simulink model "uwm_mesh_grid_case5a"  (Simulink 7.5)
settings: Solver=ode45  StartTime=0.0  StopTime=3.0  RelTol=1e-4
undefined symbols (not defined in the file or in its folder): D1, Delta, dfilt, DiscIntNeverNeededParam, Discrete, no, powergui, steady, ZData
libraries: powerlib x259, powerlib_extras x68, dsparch4 x11
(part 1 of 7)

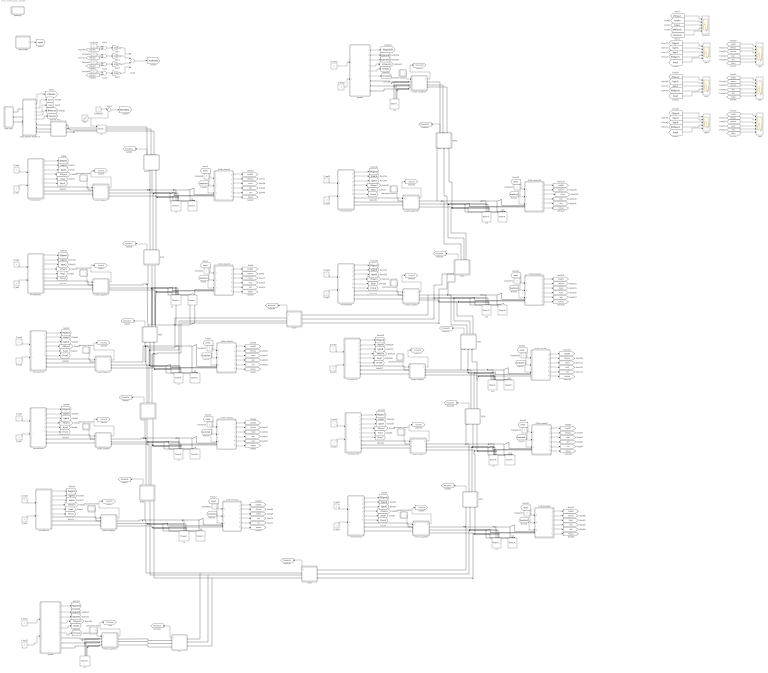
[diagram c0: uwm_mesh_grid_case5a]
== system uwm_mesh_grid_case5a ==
  2 kW e-board5 : Subsystem
  2 kW e-board9 : Subsystem
  4 kW e-board1 : Subsystem
  4 kW e-board10 : Subsystem
  4 kW e-board2 : Subsystem
  4 kW e-board3 : Subsystem
  4 kW e-board4 : Subsystem
  4 kW e-board6 : Subsystem
  4 kW e-board7 : Subsystem
  4 kW e-board8 : Subsystem
  Constant{1..3,9..15} (10 alike) : Constant  Value=2  OutDataType=fixdt(1, 16)  OutScaling=2^0
  Constant{4..8} (5 alike) : Constant  OutDataType=fixdt(1, 16)  OutScaling=2^0
  EB1 : Scope  NumInputPorts=6
  EB5 : Scope  NumInputPorts=6
  EBA : Scope  NumInputPorts=6
  E_req{1,3,5,7,9} (5 alike) : Constant  Value=.3  OutDataType=fixdt(1, 16)  OutScaling=2^0
  E_req{2,4,6,8,10,12,14,16,18,20..22} (12 alike) : Constant  OutDataType=fixdt(1, 16)  OutScaling=2^0
  E_req{11,13,15,17,19} (5 alike) : Constant  Value=.2  OutDataType=fixdt(1, 16)  OutScaling=2^0
  E_req23 : Constant  Value=.8  OutDataType=fixdt(1, 16)  OutScaling=2^0
  E_req24 : Constant  Value=.8  OutDataType=fixdt(1, 16)  OutScaling=2^0
  Gain{,1..3} (4 alike) : Gain  Gain=2/15  ParameterDataType=fixdt(1, 16)  ParameterScaling=2^0  OutDataType=fixdt(1, 16)  OutScaling=2^0
  L{1..20} (20 alike) : powerlib/Elements/Three-Phase Series RLC Load  DialogController=POWERSYS.PowerSysDialog  PhysicalDomain=powersysdomain  SubClassName=unknown  LeftPortType=p1  RightPortType=p1  LConnTagsString=A|B|C  Configuration=Y (grounded)  NominalVoltage=208  NominalFrequency=60  ActivePower=4000  InductivePower=0  CapacitivePower=0  Measurements=None
  L21 : powerlib/Elements/Three-Phase Series RLC Load  DialogController=POWERSYS.PowerSysDialog  PhysicalDomain=powersysdomain  SubClassName=unknown  LeftPortType=p1  RightPortType=p1  LConnTagsString=A|B|C  Configuration=Y (grounded)  NominalVoltage=208  NominalFrequency=60  ActivePower=8000  InductivePower=0  CapacitivePower=0  Measurements=None
  L22 : powerlib/Elements/Three-Phase Series RLC Load  DialogController=POWERSYS.PowerSysDialog  PhysicalDomain=powersysdomain  SubClassName=unknown  LeftPortType=p1  RightPortType=p1  LConnTagsString=A|B|C  Configuration=Y (grounded)  NominalVoltage=208  NominalFrequency=60  ActivePower=8000  InductivePower=0  CapacitivePower=0  Measurements=None
  MainGrid : Scope  NumInputPorts=5
  PC01 : Subsystem  mask{R=0.027352, L=.006600, C=288.6}
  PC1 : Subsystem  mask{R=0.027352, L=.006600, C=288.6}
  PC12 : Subsystem  mask{R=0.027352, L=.006600, C=288.6}
  PC2 : Subsystem  mask{R=.002810, L=.000679, C=2894.3}
  PC23 : Subsystem  mask{R=0.027352, L=.006600, C=288.6}
  PC34 : Subsystem  mask{R=0.027352, L=.006600, C=288.6}
  PC39 : Subsystem  mask{R=0.027352, L=.006600, C=288.6}
  PC45 : Subsystem  mask{R=0.027352, L=.006600, C=288.6}
  PC56 : Subsystem  mask{R=0.027352, L=.006600, C=288.6}
  PC67 : Subsystem  mask{R=0.027352, L=.006600, C=288.6}
  PC78 : Subsystem  mask{R=0.027352, L=.006600, C=288.6}
  PC89 : Subsystem  mask{R=0.027352, L=.006600, C=288.6}
  PC9A : Subsystem  mask{R=0.027352, L=.006600, C=288.6}
  PC9A1 : Subsystem  mask{R=0.027352, L=.006600, C=288.6}
  SS : powerlib/Elements/Three-Phase Breaker  DialogController=POWERSYS.PowerSysDialog  SystemSampleTime=-1  InitialState=closed  SwitchA=on  SwitchB=on  SwitchC=on  SwitchTimes=[1.]  External=on  BreakerResistance=.001  SnubberResistance=1e6  SnubberCapacitance=inf  Measurements=None
  Step : Step  Time=2  Before=1  After=0  SampleTime=0
  Sum{1..3,5} (4 alike) : Sum  Inputs=+-  OutDataType=fixdt(1, 16)  OutScaling=2^0
  Sum4 : Sum  Inputs=|+-  OutDataType=fixdt(1, 16)  OutScaling=2^0
  Sum6 : Sum  Inputs=++++  OutDataType=fixdt(1, 16)  OutScaling=2^0
  disconnect event : Subsystem  mask{tstart=50, tstop=60}
      mask prompts: tstart "disconnect time"; tstop "connect time"
  disconnect event1 : Subsystem  mask{tstart=100, tstop=200}
      mask prompts: tstart "disconnect time"; tstop "connect time"
  disconnect event10 : Subsystem  mask{tstart=100, tstop=200}
      mask prompts: tstart "disconnect time"; tstop "connect time"
  disconnect event11 : Subsystem  mask{tstart=50, tstop=60}
      mask prompts: tstart "disconnect time"; tstop "connect time"
  disconnect event2 : Subsystem  mask{tstart=100, tstop=200}
      mask prompts: tstart "disconnect time"; tstop "connect time"
  disconnect event3 : Subsystem  mask{tstart=100, tstop=200}
      mask prompts: tstart "disconnect time"; tstop "connect time"
  disconnect event4 : Subsystem  mask{tstart=100, tstop=200}
      mask prompts: tstart "disconnect time"; tstop "connect time"
  disconnect event5 : Subsystem  mask{tstart=100, tstop=200}
      mask prompts: tstart "disconnect time"; tstop "connect time"
  disconnect event6 : Subsystem  mask{tstart=100, tstop=200}
      mask prompts: tstart "disconnect time"; tstop "connect time"
  disconnect event7 : Subsystem  mask{tstart=100, tstop=200}
      mask prompts: tstart "disconnect time"; tstop "connect time"
  disconnect event8 : Subsystem  mask{tstart=100, tstop=200}
      mask prompts: tstart "disconnect time"; tstop "connect time"
  disconnect event9 : Subsystem  mask{tstart=100, tstop=200}
      mask prompts: tstart "disconnect time"; tstop "connect time"
  gen1 : Scope  NumInputPorts=5
  gen5 : Scope  NumInputPorts=5
  genA : Scope  NumInputPorts=5
  genset : Subsystem
  genset1 : Subsystem
  main grid : Subsystem
  measurement feeder C3 : Subsystem
  microsource : Subsystem  AncestorBlock=|
      | UWM_blocks/inverter-based
      | DG (simplified)
      | 208V - 15kVA
  microsource1 : Subsystem  AncestorBlock=|
      | UWM_blocks/inverter-based
      | DG (simplified)
      | 208V - 15kVA
  microsource2 : Subsystem  AncestorBlock=|
      | UWM_blocks/inverter-based
      | DG (simplified)
      | 208V - 15kVA
  microsource3 : Subsystem  AncestorBlock=|
      | UWM_blocks/inverter-based
      | DG (simplified)
      | 208V - 15kVA
  microsource4 : Subsystem  AncestorBlock=|
      | UWM_blocks/inverter-based
      | DG (simplified)
      | 208V - 15kVA
  microsource5 : Subsystem  AncestorBlock=|
      | UWM_blocks/inverter-based
      | DG (simplified)
      | 208V - 15kVA
  microsource6 : Subsystem  AncestorBlock=|
      | UWM_blocks/inverter-based
      | DG (simplified)
      | 208V - 15kVA
  microsource7 : Subsystem  AncestorBlock=|
      | UWM_blocks/inverter-based
      | DG (simplified)
      | 208V - 15kVA
  microsource8 : Subsystem  AncestorBlock=|
      | UWM_blocks/inverter-based
      | DG (simplified)
      | 208V - 15kVA
  microsource9 : Subsystem  AncestorBlock=|
      | UWM_blocks/inverter-based
      | DG (simplified)
      | 208V - 15kVA
  powergui : Subsystem  Priority=1  AncestorBlock=powerlib/powergui  InitFcn=powergui( 'InitFcn_Callback' , gcb , 0 , [ ] );  StopFcn=powergui( 'StopFcn_Callback' , gcb , 0 , [ ] );  mask(PSB option menu block){SimulationMode=Discrete, SampleTime=20e-6, frequency=60, SPID=off, DisableSnubberDevices=off, DisableRonSwitches=off, DisableVfSwitches=off, SwTol=0, Interpol=off, frequencyindice=60, echomessages=off, HookPort=off, DisplayEquations=off, FunctionMessages=off, EnableUseOfTLC=off, x0status=steady, RestoreLinks=no, ResistiveCurrentMeasurement=off, Frange=[0:2:500], Ylog=off, Xlog=on, ShowGrid=off, save=off, variable=ZData, structure=, ZoomFFT=on, StartTime=0.0, cycles=1, DisplayStyle=1, fundamental=60, FreqAxis=off, MaxFrequency=1000, frequencyindicesteady=1, RmsSteady=2, display=off, Ts=0, methode=off}
      mask prompts: SimulationMode "Simulation type:"; SampleTime "Sample time (s):"; frequency "Phasor frequency (Hz):"; SPID "Enable use of ideal switching devices"; DisableSnubberDevices "Disable snubbers in switching devices"; DisableRonSwitches "Disable On resistance in switching devices (Ron=0)"; DisableVfSwitches "Disable Forward voltage in switching devices (Vf=0)"; SwTol "Switch tolerance"; Interpol "Interpolate"; frequencyindice "Load flow frequency (Hz):"; echomessages "Display SimPowerSystems warnings and messages"; HookPort "Add a hook port to the powergui block"; DisplayEquations "Display circuit differential equations"; FunctionMessages "Display internal function messages (debug mode feature)"; EnableUseOfTLC "Use TLC file when in Accelerator Simulation Mode and for RTW applications"; x0status "Start simulation with initial electrical states from:"; RestoreLinks "Restore disabled links of SimPowerSystems blocks:"; ResistiveCurrentMeasurement "Use non ideal current measurement blocks (1e-4Ohm internal resistance)"; Frange "Frequency Range"; Ylog "Log impedance"; Xlog "log Frequency"; ShowGrid "grid"; save "Save Data To Workspace"; variable "Variable Name"; structure "Structure Name (PSBFFTSCOPE)"; ZoomFFT "ZoomFFT (PSBFFTSCOPE)"; StartTime "Start Time (PSBFFTSCOPE)"; cycles "Cycles (PSBFFTSCOPE)"; DisplayStyle "Display style (PSBFFTSCOPE)"; fundamental "Fundamental (PSBFFTSCOPE)"; FreqAxis "Frequency Axis (PSBFFTSCOPE)"; MaxFrequency "Max Frequency (PSBFFTSCOPE)"; frequencyindicesteady "Frequency indice (STEADYSTATE)"; RmsSteady "RMS display (STEADYSTATE)"; display "Display Results"; Ts "Old Ts setting (OBSOLETE)"; methode "Phasor simulation (OBSOLETE)"
      mask help: Set simulation type, simulation parameters, and preferences
      mask init:
      | message = powergui('MaskInitialization',gcb,SimulationMode,SampleTime);
  reset pulses : Subsystem  mask{tpulse=[50 100]}
  smart coupler1 : Subsystem
  smart coupler10 : Subsystem
  smart coupler11 : Subsystem
  smart coupler12 : Subsystem
  smart coupler2 : Subsystem
  smart coupler3 : Subsystem
  smart coupler4 : Subsystem
  smart coupler5 : Subsystem
  smart coupler6 : Subsystem
  smart coupler7 : Subsystem
  smart coupler8 : Subsystem
  smart coupler9 : Subsystem
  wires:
  E_req1/1 -> microsource/2(P_req)
  E_req2/1 -> microsource/1(E_req)
  reset pulses/1(Out1) -> [reset]
  4 kW e-board1/1(w) -> [freqEB1]
  4 kW e-board1/2(state) -> [EB1state]
  measurement feeder C3/3(I) -> [Imain]
  measurement feeder C3/1(PQ) -> [PQmain]
  measurement feeder C3/2(V) -> [Vmain]
  [PQmain] -> MainGrid/1
  [Vmain] -> MainGrid/2
  [Imain] -> MainGrid/3
  [RMSmain] -> MainGrid/4
  microsource/1(PQ) -> [PQgen1]
  microsource/2(V) -> [Vgen1]
  microsource/3(I) -> [Igen1]
  microsource/5(freq) -> [freq1]
  measurement feeder C3/4(RMS) -> [RMSmain]
  microsource/4(RMS) -> [RMSgen1]
  measurement feeder C3/5(freq) -> [freqmain]
  [freqmain] -> MainGrid/5
  [freqEB1] -> EB1/1
  [RMSeb1] -> EB1/2
  [EB1state] -> EB1/3
  4 kW e-board1/3(PQ) -> [PQeb1]
  4 kW e-board1/4(V) -> [Veb1]
  4 kW e-board1/5(I) -> [Ieb1]
  4 kW e-board1/6(RMS) -> [RMSeb1]
  [PQeb1] -> EB1/6
  [Ieb1] -> EB1/5
  [Veb1] -> EB1/4
  Step/1 -> SS/1, Sum4/2
  Constant5/1 -> Sum4/1
  Sum4/1 -> [IslandState]
  disconnect event1/1(Out1) -> smart coupler1/1(event)
  smart coupler1/1(connected) -> [connect1]
  Constant4/1 -> Sum1/1
  [EB1state] -> Sum1/2
  Constant6/1 -> Sum2/1
  [EB2state] -> Sum2/2
  Constant7/1 -> Sum3/1
  [EB3state] -> Sum3/2
  Constant8/1 -> Sum5/1
  [EB4state] -> Sum5/2
  Sum1/1 -> Gain/1
  Sum2/1 -> Gain1/1
  Sum3/1 -> Gain3/1
  Sum5/1 -> Gain2/1
  Gain1/1 -> Sum6/2
  Gain3/1 -> Sum6/3
  Gain/1 -> Sum6/1
  Gain2/1 -> Sum6/4
  Sum6/1 -> [loadshed]
  [reset] -> 4 kW e-board1/1(reset)
  Constant9/1 -> 4 kW e-board1/2(priority)
  [loadshed] -> 4 kW e-board1/3(shed_load)
  PC01/1(PQ) -> [PQcable01]
  microsource/6(Pmm) -> [Pmm1]
  [PQgen1] -> gen1/1
  [Vgen1] -> gen1/2
  [Igen1] -> gen1/3
  [RMSgen1] -> gen1/4
  [freq1] -> gen1/5
  E_req3/1 -> microsource1/2(P_req)
  E_req4/1 -> microsource1/1(E_req)
  4 kW e-board2/1(w) -> [freqEB2]
  4 kW e-board2/2(state) -> [EB2state]
  microsource1/1(PQ) -> [PQgen2]
  microsource1/2(V) -> [Vgen2]
  microsource1/3(I) -> [Igen2]
  microsource1/5(freq) -> [freq2]
  microsource1/4(RMS) -> [RMSgen2]
  4 kW e-board2/3(PQ) -> [PQeb2]
  4 kW e-board2/4(V) -> [Veb2]
  4 kW e-board2/5(I) -> [Ieb2]
  4 kW e-board2/6(RMS) -> [RMSeb2]
  disconnect event2/1(Out1) -> smart coupler2/1(event)
  smart coupler2/1(connected) -> [connect2]
  [reset] -> 4 kW e-board2/1(reset)
  Constant1/1 -> 4 kW e-board2/2(priority)
  [loadshed] -> 4 kW e-board2/3(shed_load)
  PC12/1(PQ) -> [PQcable12]
  microsource1/6(Pmm) -> [Pmm2]
  E_req5/1 -> microsource2/2(P_req)
  E_req6/1 -> microsource2/1(E_req)
  4 kW e-board3/1(w) -> [freqEB3]
  4 kW e-board3/2(state) -> [EB3state]
  microsource2/1(PQ) -> [PQgen3]
  microsource2/2(V) -> [Vgen3]
  microsource2/3(I) -> [Igen3]
  microsource2/5(freq) -> [freq3]
  microsource2/4(RMS) -> [RMSgen3]
  4 kW e-board3/3(PQ) -> [PQeb3]
  4 kW e-board3/4(V) -> [Veb3]
  4 kW e-board3/5(I) -> [Ieb3]
  4 kW e-board3/6(RMS) -> [RMSeb3]
  disconnect event3/1(Out1) -> smart coupler3/1(event)
  smart coupler3/1(connected) -> [connect3]
  [reset] -> 4 kW e-board3/1(reset)
  Constant2/1 -> 4 kW e-board3/2(priority)
  [loadshed] -> 4 kW e-board3/3(shed_load)
  PC23/1(PQ) -> [PQcable23]
  microsource2/6(Pmm) -> [Pmm3]
  E_req7/1 -> microsource3/2(P_req)
  E_req8/1 -> microsource3/1(E_req)
  4 kW e-board4/1(w) -> [freqEB4]
  4 kW e-board4/2(state) -> [EB4state]
  microsource3/1(PQ) -> [PQgen4]
  microsource3/2(V) -> [Vgen4]
  microsource3/3(I) -> [Igen4]
  microsource3/5(freq) -> [freq4]
  microsource3/4(RMS) -> [RMSgen4]
  4 kW e-board4/3(PQ) -> [PQeb4]
  4 kW e-board4/4(V) -> [Veb4]
  4 kW e-board4/5(I) -> [Ieb4]
  4 kW e-board4/6(RMS) -> [RMSeb4]
  disconnect event4/1(Out1) -> smart coupler4/1(event)
  smart coupler4/1(connected) -> [connect4]
  [reset] -> 4 kW e-board4/1(reset)
  Constant3/1 -> 4 kW e-board4/2(priority)
  [loadshed] -> 4 kW e-board4/3(shed_load)
  PC34/1(PQ) -> [PQcable34]
  microsource3/6(Pmm) -> [Pmm4]
  E_req9/1 -> microsource4/2(P_req)
  E_req10/1 -> microsource4/1(E_req)
  2 kW e-board5/1(w) -> [freqEB5]
  2 kW e-board5/2(state) -> [EB5state]
  microsource4/1(PQ) -> [PQgen5]
  microsource4/2(V) -> [Vgen5]
  microsource4/3(I) -> [Igen5]
  microsource4/5(freq) -> [freq5]
  microsource4/4(RMS) -> [RMSgen5]
  2 kW e-board5/3(PQ) -> [PQeb5]
  2 kW e-board5/4(V) -> [Veb5]
  2 kW e-board5/5(I) -> [Ieb5]
  2 kW e-board5/6(RMS) -> [RMSeb5]
  disconnect event5/1(Out1) -> smart coupler5/1(event)
  smart coupler5/1(connected) -> [connect5]
  [reset] -> 2 kW e-board5/1(reset)
  Constant10/1 -> 2 kW e-board5/2(priority)
  [loadshed] -> 2 kW e-board5/3(shed_load)
  PC45/1(PQ) -> [PQcable45]
  microsource4/6(Pmm) -> [Pmm5]
  E_req11/1 -> microsource5/2(P_req)
  E_req12/1 -> microsource5/1(E_req)
  4 kW e-board6/1(w) -> [freqEB6]
  4 kW e-board6/2(state) -> [EB6state]
  microsource5/1(PQ) -> [PQgen6]
  microsource5/2(V) -> [Vgen6]
  microsource5/3(I) -> [Igen6]
  microsource5/5(freq) -> [freq6]
  microsource5/4(RMS) -> [RMSgen6]
  4 kW e-board6/3(PQ) -> [PQeb6]
  4 kW e-board6/4(V) -> [Veb6]
  4 kW e-board6/5(I) -> [Ieb6]
  4 kW e-board6/6(RMS) -> [RMSeb6]
  disconnect event6/1(Out1) -> smart coupler6/1(event)
  smart coupler6/1(connected) -> [connect6]
  [reset] -> 4 kW e-board6/1(reset)
  Constant11/1 -> 4 kW e-board6/2(priority)
  [loadshed] -> 4 kW e-board6/3(shed_load)
  PC67/1(PQ) -> [PQcable67]
  microsource5/6(Pmm) -> [Pmm6]
  E_req13/1 -> microsource6/2(P_req)
  E_req14/1 -> microsource6/1(E_req)
  4 kW e-board7/1(w) -> [freqEB7]
  4 kW e-board7/2(state) -> [EB7state]
  microsource6/1(PQ) -> [PQgen7]
  microsource6/2(V) -> [Vgen7]
  microsource6/3(I) -> [Igen7]
  microsource6/5(freq) -> [freq7]
  microsource6/4(RMS) -> [RMSgen7]
  4 kW e-board7/3(PQ) -> [PQeb7]
  4 kW e-board7/4(V) -> [Veb7]
  4 kW e-board7/5(I) -> [Ieb7]
  4 kW e-board7/6(RMS) -> [RMSeb7]
  disconnect event7/1(Out1) -> smart coupler7/1(event)
  smart coupler7/1(connected) -> [connect7]
  [reset] -> 4 kW e-board7/1(reset)
  Constant12/1 -> 4 kW e-board7/2(priority)
  [loadshed] -> 4 kW e-board7/3(shed_load)
  PC78/1(PQ) -> [PQcable78]
  microsource6/6(Pmm) -> [Pmm7]
  E_req15/1 -> microsource7/2(P_req)
  E_req16/1 -> microsource7/1(E_req)
  4 kW e-board8/1(w) -> [freqEB8]
  4 kW e-board8/2(state) -> [EB8state]
  microsource7/1(PQ) -> [PQgen8]
  microsource7/2(V) -> [Vgen8]
  microsource7/3(I) -> [Igen8]
  microsource7/5(freq) -> [freq8]
  microsource7/4(RMS) -> [RMSgen8]
  4 kW e-board8/3(PQ) -> [PQeb8]
  4 kW e-board8/4(V) -> [Veb8]
  4 kW e-board8/5(I) -> [Ieb8]
  4 kW e-board8/6(RMS) -> [RMSeb8]
  disconnect event8/1(Out1) -> smart coupler8/1(event)
  smart coupler8/1(connected) -> [connect8]
  [reset] -> 4 kW e-board8/1(reset)
  Constant13/1 -> 4 kW e-board8/2(priority)
  [loadshed] -> 4 kW e-board8/3(shed_load)
  PC89/1(PQ) -> [PQcable89]
  microsource7/6(Pmm) -> [Pmm8]
  E_req17/1 -> microsource8/2(P_req)
  E_req18/1 -> microsource8/1(E_req)
  2 kW e-board9/1(w) -> [freqEB9]
  2 kW e-board9/2(state) -> [EB9state]
  microsource8/1(PQ) -> [PQgen9]
  microsource8/2(V) -> [Vgen9]
  microsource8/3(I) -> [Igen9]
  microsource8/5(freq) -> [freq9]
  microsource8/4(RMS) -> [RMSgen9]
  2 kW e-board9/3(PQ) -> [PQeb9]
  2 kW e-board9/4(V) -> [Veb9]
  2 kW e-board9/5(I) -> [Ieb9]
  2 kW e-board9/6(RMS) -> [RMSeb9]
  disconnect event9/1(Out1) -> smart coupler9/1(event)
  smart coupler9/1(connected) -> [connect9]
  [reset] -> 2 kW e-board9/1(reset)
  Constant14/1 -> 2 kW e-board9/2(priority)
  [loadshed] -> 2 kW e-board9/3(shed_load)
  PC9A/1(PQ) -> [PQcable9A]
  microsource8/6(Pmm) -> [Pmm9]
  E_req19/1 -> microsource9/2(P_req)
  E_req20/1 -> microsource9/1(E_req)
  4 kW e-board10/1(w) -> [freqEBA]
  4 kW e-board10/2(state) -> [EBAstate]
  microsource9/1(PQ) -> [PQgenA]
  microsource9/2(V) -> [VgenA]
  microsource9/3(I) -> [IgenA]
  microsource9/5(freq) -> [freqA]
  microsource9/4(RMS) -> [RMSgenA]
  4 kW e-board10/3(PQ) -> [PQebA]
  4 kW e-board10/4(V) -> [VebA]
  4 kW e-board10/5(I) -> [IebA]
  4 kW e-board10/6(RMS) -> [RMSebA]
  disconnect event10/1(Out1) -> smart coupler10/1(event)
  smart coupler10/1(connected) -> [connectA]
  [reset] -> 4 kW e-board10/1(reset)
  Constant15/1 -> 4 kW e-board10/2(priority)
  [loadshed] -> 4 kW e-board10/3(shed_load)
  microsource9/6(Pmm) -> [PmmA]
  PC56/1(PQ) -> [PQcable56]
  [freqEB5] -> EB5/1
  [RMSeb5] -> EB5/2
  [EB5state] -> EB5/3
  [PQeb5] -> EB5/6
  [Ieb5] -> EB5/5
  [Veb5] -> EB5/4
  [PQgen5] -> gen5/1
  [Vgen5] -> gen5/2
  [Igen5] -> gen5/3
  [RMSgen5] -> gen5/4
  [freq5] -> gen5/5
  [freqEBA] -> EBA/1
  [RMSebA] -> EBA/2
  [EBAstate] -> EBA/3
  [PQebA] -> EBA/6
  [IebA] -> EBA/5
  [VebA] -> EBA/4
  [PQgenA] -> genA/1
  [VgenA] -> genA/2
  [IgenA] -> genA/3
  [RMSgenA] -> genA/4
  [freqA] -> genA/5
  PC39/1(PQ) -> [PQcable39]
  E_req21/1 -> genset/1(Ereq)
  E_req23/1 -> genset/2(Preq)
  genset/1(PQ) -> [PQgenGS]
  genset/2(V) -> [VgenGS]
  genset/3(I) -> [IgenGS]
  genset/5(freq) -> [freqGS]
  genset/4(RMS) -> [RMSgenGS]
  disconnect event/1(Out1) -> smart coupler11/1(event)
  smart coupler11/1(connected) -> [GSconnect]
  genset/6(Pmm) -> [PmmGS]
  E_req22/1 -> genset1/1(Ereq)
  E_req24/1 -> genset1/2(Preq)
  genset1/1(PQ) -> [PQgenGS1]
  genset1/2(V) -> [VgenGS1]
  genset1/3(I) -> [IgenGS1]
  genset1/5(freq) -> [freqGS1]
  genset1/4(RMS) -> [RMSgenGS1]
  disconnect event11/1(Out1) -> smart coupler12/1(event)
  smart coupler12/1(connected) -> [GSconnect1]
  genset1/6(Pmm) -> [PmmGS1]
  PC1/1(PQ) -> [PQcableGS]
  PC9A1/1(PQ) -> [PQcableGS1]
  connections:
  main grid/RConn2 -- measurement feeder C3/LConn2
  main grid/RConn1 -- measurement feeder C3/LConn1
  measurement feeder C3/LConn3 -- main grid/RConn3
  measurement feeder C3/RConn1 -- PC2/LConn1
  measurement feeder C3/RConn2 -- PC2/LConn2
  measurement feeder C3/RConn3 -- PC2/LConn3
  PC2/RConn2 -- SS/LConn2
  PC2/RConn1 -- SS/LConn1
  SS/LConn3 -- PC2/RConn3
  microsource/RConn1 -- smart coupler1/LConn1
  smart coupler1/LConn2 -- microsource/RConn2
  smart coupler1/LConn3 -- microsource/RConn3
  smart coupler1/RConn1 -- PC01/LConn1 -- L3/LConn1 -- L4/LConn1 -- 4 kW e-board1/LConn1 -- PC12/RConn1
  L3/LConn2 -- L4/LConn2 -- 4 kW e-board1/LConn2 -- smart coupler1/RConn2 -- PC01/LConn2 -- PC12/RConn2
  L3/LConn3 -- L4/LConn3 -- 4 kW e-board1/LConn3 -- smart coupler1/RConn3 -- PC01/LConn3 -- PC12/RConn3
  PC23/RConn1 -- smart coupler2/RConn1 -- PC12/LConn1 -- L1/LConn1 -- L2/LConn1 -- 4 kW e-board2/LConn1
  PC23/RConn2 -- L1/LConn2 -- L2/LConn2 -- 4 kW e-board2/LConn2 -- smart coupler2/RConn2 -- PC12/LConn2
  PC23/RConn3 -- smart coupler2/RConn3 -- L1/LConn3 -- L2/LConn3 -- 4 kW e-board2/LConn3 -- PC12/LConn3
  microsource1/RConn1 -- smart coupler2/LConn1
  smart coupler2/LConn2 -- microsource1/RConn2
  smart coupler2/LConn3 -- microsource1/RConn3
  smart coupler3/RConn1 -- L5/LConn1 -- L6/LConn1 -- 4 kW e-board3/LConn1 -- PC34/RConn1 -- PC23/LConn1 -- PC39/RConn1
  L5/LConn2 -- L6/LConn2 -- 4 kW e-board3/LConn2 -- smart coupler3/RConn2 -- PC34/RConn2 -- PC23/LConn2 -- PC39/RConn2
  smart coupler3/RConn3 -- PC34/RConn3 -- L5/LConn3 -- L6/LConn3 -- 4 kW e-board3/LConn3 -- PC23/LConn3 -- PC39/RConn3
  microsource2/RConn1 -- smart coupler3/LConn1
  smart coupler3/LConn2 -- microsource2/RConn2
  smart coupler3/LConn3 -- microsource2/RConn3
  smart coupler4/RConn1 -- PC34/LConn1 -- L7/LConn1 -- L8/LConn1 -- 4 kW e-board4/LConn1 -- PC45/RConn1
  L7/LConn2 -- L8/LConn2 -- 4 kW e-board4/LConn2 -- PC34/LConn2 -- smart coupler4/RConn2 -- PC45/RConn2
  L7/LConn3 -- L8/LConn3 -- 4 kW e-board4/LConn3 -- smart coupler4/RConn3 -- PC34/LConn3 -- PC45/RConn3
  microsource3/RConn1 -- smart coupler4/LConn1
  smart coupler4/LConn2 -- microsource3/RConn2
  smart coupler4/LConn3 -- microsource3/RConn3
  PC56/RConn1 -- smart coupler5/RConn1 -- L9/LConn1 -- L10/LConn1 -- 2 kW e-board5/LConn1 -- PC45/LConn1 -- PC1/LConn1
  PC56/RConn2 -- L9/LConn2 -- L10/LConn2 -- 2 kW e-board5/LConn2 -- smart coupler5/RConn2 -- PC45/LConn2 -- PC1/LConn2
  PC56/RConn3 -- L9/LConn3 -- L10/LConn3 -- 2 kW e-board5/LConn3 -- smart coupler5/RConn3 -- PC45/LConn3 -- PC1/LConn3
  microsource4/RConn1 -- smart coupler5/LConn1
  smart coupler5/LConn2 -- microsource4/RConn2
  smart coupler5/LConn3 -- microsource4/RConn3
  smart coupler6/RConn1 -- PC56/LConn1 -- L11/LConn1 -- L12/LConn1 -- 4 kW e-board6/LConn1 -- PC67/LConn1
  L11/LConn2 -- L12/LConn2 -- 4 kW e-board6/LConn2 -- smart coupler6/RConn2 -- PC56/LConn2 -- PC67/LConn2
  L11/LConn3 -- L12/LConn3 -- 4 kW e-board6/LConn3 -- smart coupler6/RConn3 -- PC56/LConn3 -- PC67/LConn3
  microsource5/RConn1 -- smart coupler6/LConn1
  smart coupler6/LConn2 -- microsource5/RConn2
  smart coupler6/LConn3 -- microsource5/RConn3
  smart coupler7/RConn1 -- L13/LConn1 -- L14/LConn1 -- 4 kW e-board7/LConn1 -- PC67/RConn1 -- PC78/LConn1
  L13/LConn2 -- L14/LConn2 -- 4 kW e-board7/LConn2 -- smart coupler7/RConn2 -- PC67/RConn2 -- PC78/LConn2
  L13/LConn3 -- L14/LConn3 -- 4 kW e-board7/LConn3 -- smart coupler7/RConn3 -- PC67/RConn3 -- PC78/LConn3
  microsource6/RConn1 -- smart coupler7/LConn1
  smart coupler7/LConn2 -- microsource6/RConn2
  smart coupler7/LConn3 -- microsource6/RConn3
  smart coupler8/RConn1 -- L15/LConn1 -- L16/LConn1 -- 4 kW e-board8/LConn1 -- PC78/RConn1 -- PC89/LConn1
  L15/LConn2 -- L16/LConn2 -- 4 kW e-board8/LConn2 -- PC78/RConn2 -- smart coupler8/RConn2 -- PC89/LConn2
  PC78/RConn3 -- L15/LConn3 -- L16/LConn3 -- 4 kW e-board8/LConn3 -- smart coupler8/RConn3 -- PC89/LConn3
  microsource7/RConn1 -- smart coupler8/LConn1
  smart coupler8/LConn2 -- microsource7/RConn2
  smart coupler8/LConn3 -- microsource7/RConn3
  smart coupler9/RConn1 -- L17/LConn1 -- L18/LConn1 -- 2 kW e-board9/LConn1 -- PC89/RConn1 -- PC9A/LConn1 -- PC39/LConn1
  L17/LConn2 -- L18/LConn2 -- 2 kW e-board9/LConn2 -- PC89/RConn2 -- PC9A/LConn2 -- smart coupler9/RConn2 -- PC39/LConn2
  L17/LConn3 -- L18/LConn3 -- 2 kW e-board9/LConn3 -- PC89/RConn3 -- PC9A/LConn3 -- smart coupler9/RConn3 -- PC39/LConn3
  microsource8/RConn1 -- smart coupler9/LConn1
  smart coupler9/LConn2 -- microsource8/RConn2
  smart coupler9/LConn3 -- microsource8/RConn3
  smart coupler10/RConn1 -- L19/LConn1 -- L20/LConn1 -- 4 kW e-board10/LConn1 -- PC9A/RConn1 -- PC9A1/LConn1
  L19/LConn2 -- L20/LConn2 -- 4 kW e-board10/LConn2 -- smart coupler10/RConn2 -- PC9A/RConn2 -- PC9A1/LConn2
  L19/LConn3 -- L20/LConn3 -- 4 kW e-board10/LConn3 -- smart coupler10/RConn3 -- PC9A/RConn3 -- PC9A1/LConn3
  microsource9/RConn1 -- smart coupler10/LConn1
  smart coupler10/LConn2 -- microsource9/RConn2
  smart coupler10/LConn3 -- microsource9/RConn3
  SS/RConn1 -- PC01/RConn1
  SS/RConn2 -- PC01/RConn2
  SS/RConn3 -- PC01/RConn3
  smart coupler11/LConn1 -- L21/LConn1 -- genset/RConn1
  smart coupler11/LConn2 -- L21/LConn2 -- genset/RConn2
  smart coupler11/LConn3 -- L21/LConn3 -- genset/RConn3
  smart coupler12/LConn1 -- L22/LConn1 -- genset1/RConn1
  smart coupler12/LConn2 -- L22/LConn2 -- genset1/RConn2
  smart coupler12/LConn3 -- L22/LConn3 -- genset1/RConn3
  smart coupler12/RConn3 -- PC9A1/RConn3
  smart coupler12/RConn2 -- PC9A1/RConn2
  smart coupler12/RConn1 -- PC9A1/RConn1
  PC1/RConn1 -- smart coupler11/RConn1
  PC1/RConn2 -- smart coupler11/RConn2
  PC1/RConn3 -- smart coupler11/RConn3

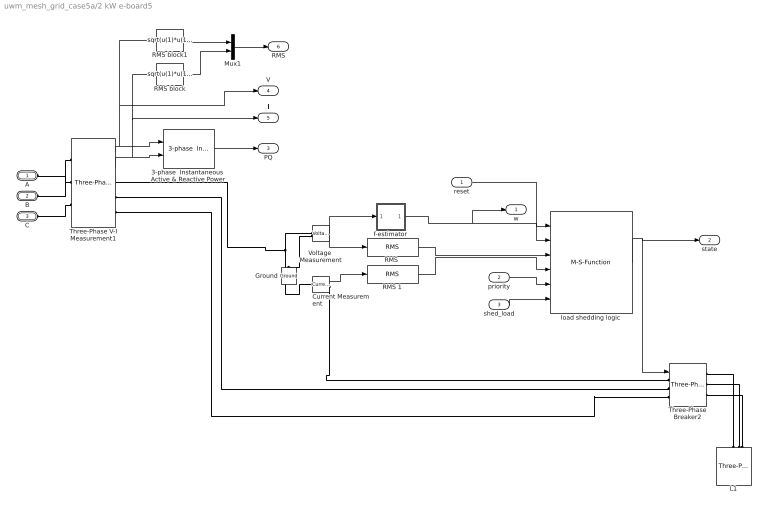
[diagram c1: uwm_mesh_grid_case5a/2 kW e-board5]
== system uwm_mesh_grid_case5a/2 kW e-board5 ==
  reset : Inport
  priority : Inport  Port=2
  shed_load : Inport  Port=3
  3-phase  Instantaneous  Active & Reactive Power : powerlib_extras/Measurements/3-phase  Instantaneous  Active & Reactive Power  DialogController=POWERSYS.PowerSysDialog  SystemSampleTime=-1
  Current Measurement : powerlib/Measurements/Current Measurement  DialogController=POWERSYS.PowerSysDialog  SystemSampleTime=-1  PhasorSimulation=off  OutputType=Complex  PSBequivalent=0
  Ground : powerlib/Elements/Ground  DialogController=POWERSYS.PowerSysDialog  PhysicalDomain=powersysdomain  SubClassName=unknown  LeftPortType=p1  RightPortType=p1  LConnTagsString=a
  L1 : powerlib/Elements/Three-Phase Series RLC Load  DialogController=POWERSYS.PowerSysDialog  PhysicalDomain=powersysdomain  SubClassName=unknown  LeftPortType=p1  RightPortType=p1  LConnTagsString=A|B|C  Configuration=Y (grounded)  NominalVoltage=208  NominalFrequency=60  ActivePower=2000  InductivePower=0  CapacitivePower=0  Measurements=None
  Mux1 : Mux  Inputs=2
  "RMS " : powerlib_extras/Measurements/RMS  DialogController=POWERSYS.PowerSysDialog  SystemSampleTime=-1  f1=60
  RMS 1 : powerlib_extras/Measurements/RMS  DialogController=POWERSYS.PowerSysDialog  SystemSampleTime=-1  f1=60
  RMS block : Fcn  Expr=sqrt(u(1)*u(1)+u(2)*u(2)+u(3)*u(3))/sqrt(3)
  RMS block1 : Fcn  Expr=sqrt(u(1)*u(1)+u(2)*u(2)+u(3)*u(3))/sqrt(3)
  Three-Phase V-I Measurement1 : powerlib/Measurements/Three-Phase V-I Measurement  DialogController=POWERSYS.PowerSysDialog  SystemSampleTime=-1  VoltageMeasurement=phase-to-ground  SetLabelV=off  LabelV=Vabc  Vpu=off  VpuLL=off  CurrentMeasurement=yes  SetLabelI=off  LabelI=Iabc  Ipu=off  Pbase=100e6  Vbase=500e3  OutputType=Complex  PhasorSimulation=off  PSBequivalent=0
  Three-Phase Breaker2 : powerlib/Elements/Three-Phase Breaker  DialogController=POWERSYS.PowerSysDialog  SystemSampleTime=-1  InitialState=closed  SwitchA=on  SwitchB=on  SwitchC=on  SwitchTimes=[50]  External=on  BreakerResistance=0.001  SnubberResistance=1e6  SnubberCapacitance=inf  Measurements=None
  Voltage  Measurement : powerlib/Measurements/Voltage Measurement  DialogController=POWERSYS.PowerSysDialog  SystemSampleTime=-1  PhasorSimulation=off  OutputType=Complex  PSBequivalent=0
  f-estimator : Subsystem  mask{dt=0.010}
      mask prompts: dt "sample time"
  load shedding logic : M-S-Function  FunctionName=load_shedding_logic3
  A : PMIOPort  Port=1  Side=Left
  B : PMIOPort  Port=2  Side=Left
  C : PMIOPort  Port=3  Side=Left
  w : Outport  OutDataType=fixdt(1, 16)  OutScaling=2^0
  state : Outport  Port=2  OutDataType=fixdt(1, 16)  OutScaling=2^0
  PQ : Outport  Port=3  OutDataType=fixdt(1, 16)  OutScaling=2^0
  V : Outport  Port=4  OutDataType=fixdt(1, 16)  OutScaling=2^0
  I : Outport  Port=5  OutDataType=fixdt(1, 16)  OutScaling=2^0
  RMS : Outport  Port=6  OutDataType=fixdt(1, 16)  OutScaling=2^0
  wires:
  reset/1 -> load shedding logic/1
  Current Measurement/1 -> RMS 1/1
  Voltage  Measurement/1 -> "RMS "/1, f-estimator/1(v)
  f-estimator/1(w) -> load shedding logic/2, w/1
  "RMS "/1 -> load shedding logic/3
  RMS 1/1 -> load shedding logic/4
  load shedding logic/1 -> Three-Phase Breaker2/1, state/1
  priority/1 -> load shedding logic/5
  Three-Phase V-I Measurement1/1 -> 3-phase  Instantaneous  Active & Reactive Power/1, RMS block1/1, V/1
  Three-Phase V-I Measurement1/2 -> 3-phase  Instantaneous  Active & Reactive Power/2, RMS block/1, I/1
  3-phase  Instantaneous  Active & Reactive Power/1 -> PQ/1
  RMS block1/1 -> Mux1/1
  RMS block/1 -> Mux1/2
  Mux1/1 -> RMS/1
  shed_load/1 -> load shedding logic/6
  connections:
  Voltage  Measurement/LConn1 -- Current Measurement/LConn1 -- Three-Phase V-I Measurement1/RConn1
  Voltage  Measurement/LConn2 -- Ground/LConn1
  Current Measurement/RConn1 -- Three-Phase Breaker2/LConn1
  L1/LConn1 -- Three-Phase Breaker2/RConn1
  L1/LConn2 -- Three-Phase Breaker2/RConn2
  L1/LConn3 -- Three-Phase Breaker2/RConn3
  Three-Phase V-I Measurement1/LConn1 -- A/RConn1
  Three-Phase V-I Measurement1/LConn2 -- B/RConn1
  Three-Phase V-I Measurement1/LConn3 -- C/RConn1
  Three-Phase V-I Measurement1/RConn2 -- Three-Phase Breaker2/LConn2
  Three-Phase V-I Measurement1/RConn3 -- Three-Phase Breaker2/LConn3

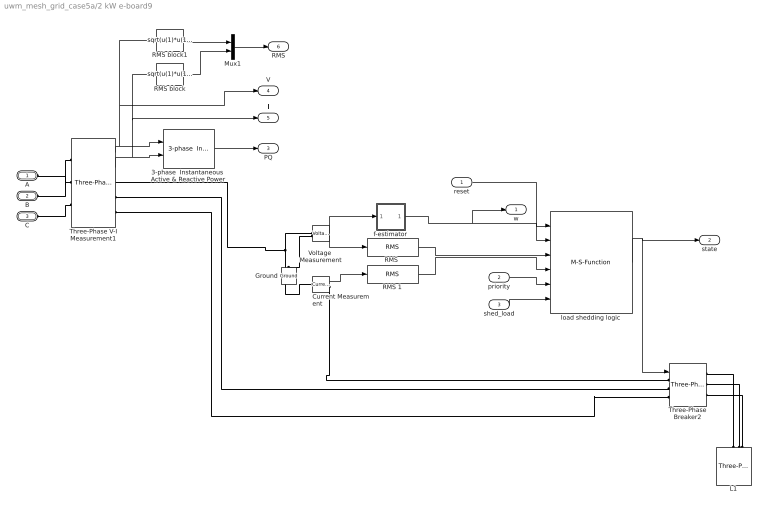
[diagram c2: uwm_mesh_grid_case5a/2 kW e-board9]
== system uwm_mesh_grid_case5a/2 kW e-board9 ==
  reset : Inport
  priority : Inport  Port=2
  shed_load : Inport  Port=3
  3-phase  Instantaneous  Active & Reactive Power : powerlib_extras/Measurements/3-phase  Instantaneous  Active & Reactive Power  DialogController=POWERSYS.PowerSysDialog  SystemSampleTime=-1
  Current Measurement : powerlib/Measurements/Current Measurement  DialogController=POWERSYS.PowerSysDialog  SystemSampleTime=-1  PhasorSimulation=off  OutputType=Complex  PSBequivalent=0
  Ground : powerlib/Elements/Ground  DialogController=POWERSYS.PowerSysDialog  PhysicalDomain=powersysdomain  SubClassName=unknown  LeftPortType=p1  RightPortType=p1  LConnTagsString=a
  L1 : powerlib/Elements/Three-Phase Series RLC Load  DialogController=POWERSYS.PowerSysDialog  PhysicalDomain=powersysdomain  SubClassName=unknown  LeftPortType=p1  RightPortType=p1  LConnTagsString=A|B|C  Configuration=Y (grounded)  NominalVoltage=208  NominalFrequency=60  ActivePower=4000  InductivePower=0  CapacitivePower=0  Measurements=None
  Mux1 : Mux  Inputs=2
  "RMS " : powerlib_extras/Measurements/RMS  DialogController=POWERSYS.PowerSysDialog  SystemSampleTime=-1  f1=60
  RMS 1 : powerlib_extras/Measurements/RMS  DialogController=POWERSYS.PowerSysDialog  SystemSampleTime=-1  f1=60
  RMS block : Fcn  Expr=sqrt(u(1)*u(1)+u(2)*u(2)+u(3)*u(3))/sqrt(3)
  RMS block1 : Fcn  Expr=sqrt(u(1)*u(1)+u(2)*u(2)+u(3)*u(3))/sqrt(3)
  Three-Phase V-I Measurement1 : powerlib/Measurements/Three-Phase V-I Measurement  DialogController=POWERSYS.PowerSysDialog  SystemSampleTime=-1  VoltageMeasurement=phase-to-ground  SetLabelV=off  LabelV=Vabc  Vpu=off  VpuLL=off  CurrentMeasurement=yes  SetLabelI=off  LabelI=Iabc  Ipu=off  Pbase=100e6  Vbase=500e3  OutputType=Complex  PhasorSimulation=off  PSBequivalent=0
  Three-Phase Breaker2 : powerlib/Elements/Three-Phase Breaker  DialogController=POWERSYS.PowerSysDialog  SystemSampleTime=-1  InitialState=closed  SwitchA=on  SwitchB=on  SwitchC=on  SwitchTimes=[50]  External=on  BreakerResistance=0.001  SnubberResistance=1e6  SnubberCapacitance=inf  Measurements=None
  Voltage  Measurement : powerlib/Measurements/Voltage Measurement  DialogController=POWERSYS.PowerSysDialog  SystemSampleTime=-1  PhasorSimulation=off  OutputType=Complex  PSBequivalent=0
  f-estimator : Subsystem  mask{dt=0.010}
      mask prompts: dt "sample time"
  load shedding logic : M-S-Function  FunctionName=load_shedding_logic3
  A : PMIOPort  Port=1  Side=Left
  B : PMIOPort  Port=2  Side=Left
  C : PMIOPort  Port=3  Side=Left
  w : Outport  OutDataType=fixdt(1, 16)  OutScaling=2^0
  state : Outport  Port=2  OutDataType=fixdt(1, 16)  OutScaling=2^0
  PQ : Outport  Port=3  OutDataType=fixdt(1, 16)  OutScaling=2^0
  V : Outport  Port=4  OutDataType=fixdt(1, 16)  OutScaling=2^0
  I : Outport  Port=5  OutDataType=fixdt(1, 16)  OutScaling=2^0
  RMS : Outport  Port=6  OutDataType=fixdt(1, 16)  OutScaling=2^0
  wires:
  reset/1 -> load shedding logic/1
  Current Measurement/1 -> RMS 1/1
  Voltage  Measurement/1 -> "RMS "/1, f-estimator/1(v)
  f-estimator/1(w) -> load shedding logic/2, w/1
  "RMS "/1 -> load shedding logic/3
  RMS 1/1 -> load shedding logic/4
  load shedding logic/1 -> Three-Phase Breaker2/1, state/1
  priority/1 -> load shedding logic/5
  Three-Phase V-I Measurement1/1 -> 3-phase  Instantaneous  Active & Reactive Power/1, RMS block1/1, V/1
  Three-Phase V-I Measurement1/2 -> 3-phase  Instantaneous  Active & Reactive Power/2, RMS block/1, I/1
  3-phase  Instantaneous  Active & Reactive Power/1 -> PQ/1
  RMS block1/1 -> Mux1/1
  RMS block/1 -> Mux1/2
  Mux1/1 -> RMS/1
  shed_load/1 -> load shedding logic/6
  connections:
  Voltage  Measurement/LConn1 -- Current Measurement/LConn1 -- Three-Phase V-I Measurement1/RConn1
  Voltage  Measurement/LConn2 -- Ground/LConn1
  Current Measurement/RConn1 -- Three-Phase Breaker2/LConn1
  L1/LConn1 -- Three-Phase Breaker2/RConn1
  L1/LConn2 -- Three-Phase Breaker2/RConn2
  L1/LConn3 -- Three-Phase Breaker2/RConn3
  Three-Phase V-I Measurement1/LConn1 -- A/RConn1
  Three-Phase V-I Measurement1/LConn2 -- B/RConn1
  Three-Phase V-I Measurement1/LConn3 -- C/RConn1
  Three-Phase V-I Measurement1/RConn2 -- Three-Phase Breaker2/LConn2
  Three-Phase V-I Measurement1/RConn3 -- Three-Phase Breaker2/LConn3

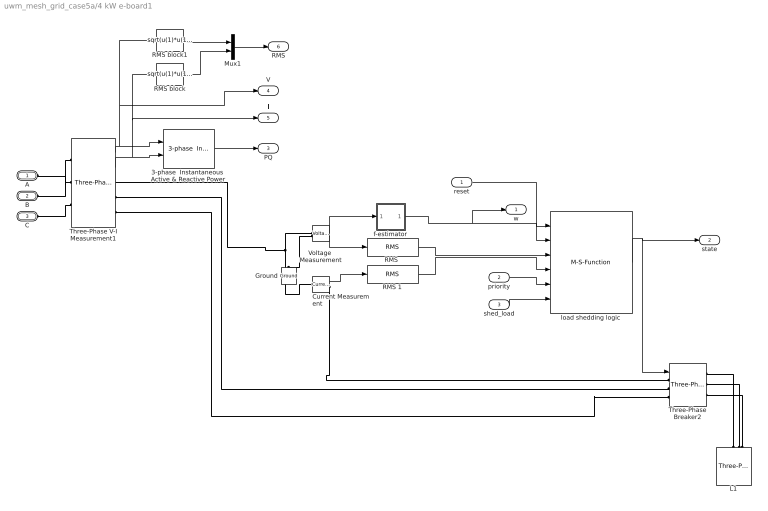
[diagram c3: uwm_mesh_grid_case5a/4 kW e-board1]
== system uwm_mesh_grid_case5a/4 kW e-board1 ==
  reset : Inport
  priority : Inport  Port=2
  shed_load : Inport  Port=3
  3-phase  Instantaneous  Active & Reactive Power : powerlib_extras/Measurements/3-phase  Instantaneous  Active & Reactive Power  DialogController=POWERSYS.PowerSysDialog  SystemSampleTime=-1
  Current Measurement : powerlib/Measurements/Current Measurement  DialogController=POWERSYS.PowerSysDialog  SystemSampleTime=-1  PhasorSimulation=off  OutputType=Complex  PSBequivalent=0
  Ground : powerlib/Elements/Ground  DialogController=POWERSYS.PowerSysDialog  PhysicalDomain=powersysdomain  SubClassName=unknown  LeftPortType=p1  RightPortType=p1  LConnTagsString=a
  L1 : powerlib/Elements/Three-Phase Series RLC Load  DialogController=POWERSYS.PowerSysDialog  PhysicalDomain=powersysdomain  SubClassName=unknown  LeftPortType=p1  RightPortType=p1  LConnTagsString=A|B|C  Configuration=Y (grounded)  NominalVoltage=208  NominalFrequency=60  ActivePower=4000  InductivePower=0  CapacitivePower=0  Measurements=None
  Mux1 : Mux  Inputs=2
  "RMS " : powerlib_extras/Measurements/RMS  DialogController=POWERSYS.PowerSysDialog  SystemSampleTime=-1  f1=60
  RMS 1 : powerlib_extras/Measurements/RMS  DialogController=POWERSYS.PowerSysDialog  SystemSampleTime=-1  f1=60
  RMS block : Fcn  Expr=sqrt(u(1)*u(1)+u(2)*u(2)+u(3)*u(3))/sqrt(3)
  RMS block1 : Fcn  Expr=sqrt(u(1)*u(1)+u(2)*u(2)+u(3)*u(3))/sqrt(3)
  Three-Phase V-I Measurement1 : powerlib/Measurements/Three-Phase V-I Measurement  DialogController=POWERSYS.PowerSysDialog  SystemSampleTime=-1  VoltageMeasurement=phase-to-ground  SetLabelV=off  LabelV=Vabc  Vpu=off  VpuLL=off  CurrentMeasurement=yes  SetLabelI=off  LabelI=Iabc  Ipu=off  Pbase=100e6  Vbase=500e3  OutputType=Complex  PhasorSimulation=off  PSBequivalent=0
  Three-Phase Breaker2 : powerlib/Elements/Three-Phase Breaker  DialogController=POWERSYS.PowerSysDialog  SystemSampleTime=-1  InitialState=closed  SwitchA=on  SwitchB=on  SwitchC=on  SwitchTimes=[50]  External=on  BreakerResistance=0.001  SnubberResistance=1e6  SnubberCapacitance=inf  Measurements=None
  Voltage  Measurement : powerlib/Measurements/Voltage Measurement  DialogController=POWERSYS.PowerSysDialog  SystemSampleTime=-1  PhasorSimulation=off  OutputType=Complex  PSBequivalent=0
  f-estimator : Subsystem  mask{dt=0.010}
      mask prompts: dt "sample time"
  load shedding logic : M-S-Function  FunctionName=load_shedding_logic3
  A : PMIOPort  Port=1  Side=Left
  B : PMIOPort  Port=2  Side=Left
  C : PMIOPort  Port=3  Side=Left
  w : Outport  OutDataType=fixdt(1, 16)  OutScaling=2^0
  state : Outport  Port=2  OutDataType=fixdt(1, 16)  OutScaling=2^0
  PQ : Outport  Port=3  OutDataType=fixdt(1, 16)  OutScaling=2^0
  V : Outport  Port=4  OutDataType=fixdt(1, 16)  OutScaling=2^0
  I : Outport  Port=5  OutDataType=fixdt(1, 16)  OutScaling=2^0
  RMS : Outport  Port=6  OutDataType=fixdt(1, 16)  OutScaling=2^0
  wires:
  reset/1 -> load shedding logic/1
  Current Measurement/1 -> RMS 1/1
  Voltage  Measurement/1 -> "RMS "/1, f-estimator/1(v)
  f-estimator/1(w) -> load shedding logic/2, w/1
  "RMS "/1 -> load shedding logic/3
  RMS 1/1 -> load shedding logic/4
  load shedding logic/1 -> Three-Phase Breaker2/1, state/1
  priority/1 -> load shedding logic/5
  Three-Phase V-I Measurement1/1 -> 3-phase  Instantaneous  Active & Reactive Power/1, RMS block1/1, V/1
  Three-Phase V-I Measurement1/2 -> 3-phase  Instantaneous  Active & Reactive Power/2, RMS block/1, I/1
  3-phase  Instantaneous  Active & Reactive Power/1 -> PQ/1
  RMS block1/1 -> Mux1/1
  RMS block/1 -> Mux1/2
  Mux1/1 -> RMS/1
  shed_load/1 -> load shedding logic/6
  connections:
  Voltage  Measurement/LConn1 -- Current Measurement/LConn1 -- Three-Phase V-I Measurement1/RConn1
  Voltage  Measurement/LConn2 -- Ground/LConn1
  Current Measurement/RConn1 -- Three-Phase Breaker2/LConn1
  L1/LConn1 -- Three-Phase Breaker2/RConn1
  L1/LConn2 -- Three-Phase Breaker2/RConn2
  L1/LConn3 -- Three-Phase Breaker2/RConn3
  Three-Phase V-I Measurement1/LConn1 -- A/RConn1
  Three-Phase V-I Measurement1/LConn2 -- B/RConn1
  Three-Phase V-I Measurement1/LConn3 -- C/RConn1
  Three-Phase V-I Measurement1/RConn2 -- Three-Phase Breaker2/LConn2
  Three-Phase V-I Measurement1/RConn3 -- Three-Phase Breaker2/LConn3

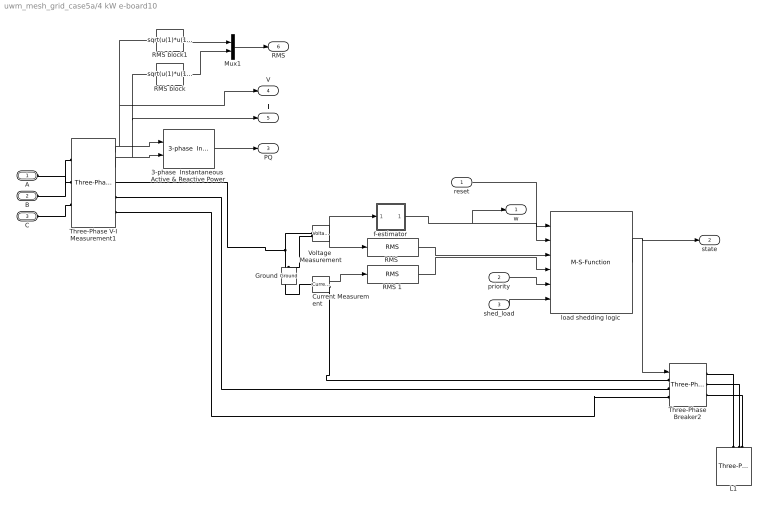
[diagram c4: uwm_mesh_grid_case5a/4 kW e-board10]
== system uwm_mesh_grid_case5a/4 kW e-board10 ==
  reset : Inport
  priority : Inport  Port=2
  shed_load : Inport  Port=3
  3-phase  Instantaneous  Active & Reactive Power : powerlib_extras/Measurements/3-phase  Instantaneous  Active & Reactive Power  DialogController=POWERSYS.PowerSysDialog  SystemSampleTime=-1
  Current Measurement : powerlib/Measurements/Current Measurement  DialogController=POWERSYS.PowerSysDialog  SystemSampleTime=-1  PhasorSimulation=off  OutputType=Complex  PSBequivalent=0
  Ground : powerlib/Elements/Ground  DialogController=POWERSYS.PowerSysDialog  PhysicalDomain=powersysdomain  SubClassName=unknown  LeftPortType=p1  RightPortType=p1  LConnTagsString=a
  L1 : powerlib/Elements/Three-Phase Series RLC Load  DialogController=POWERSYS.PowerSysDialog  PhysicalDomain=powersysdomain  SubClassName=unknown  LeftPortType=p1  RightPortType=p1  LConnTagsString=A|B|C  Configuration=Y (grounded)  NominalVoltage=208  NominalFrequency=60  ActivePower=4000  InductivePower=0  CapacitivePower=0  Measurements=None
  Mux1 : Mux  Inputs=2
  "RMS " : powerlib_extras/Measurements/RMS  DialogController=POWERSYS.PowerSysDialog  SystemSampleTime=-1  f1=60
  RMS 1 : powerlib_extras/Measurements/RMS  DialogController=POWERSYS.PowerSysDialog  SystemSampleTime=-1  f1=60
  RMS block : Fcn  Expr=sqrt(u(1)*u(1)+u(2)*u(2)+u(3)*u(3))/sqrt(3)
  RMS block1 : Fcn  Expr=sqrt(u(1)*u(1)+u(2)*u(2)+u(3)*u(3))/sqrt(3)
  Three-Phase V-I Measurement1 : powerlib/Measurements/Three-Phase V-I Measurement  DialogController=POWERSYS.PowerSysDialog  SystemSampleTime=-1  VoltageMeasurement=phase-to-ground  SetLabelV=off  LabelV=Vabc  Vpu=off  VpuLL=off  CurrentMeasurement=yes  SetLabelI=off  LabelI=Iabc  Ipu=off  Pbase=100e6  Vbase=500e3  OutputType=Complex  PhasorSimulation=off  PSBequivalent=0
  Three-Phase Breaker2 : powerlib/Elements/Three-Phase Breaker  DialogController=POWERSYS.PowerSysDialog  SystemSampleTime=-1  InitialState=closed  SwitchA=on  SwitchB=on  SwitchC=on  SwitchTimes=[50]  External=on  BreakerResistance=0.001  SnubberResistance=1e6  SnubberCapacitance=inf  Measurements=None
  Voltage  Measurement : powerlib/Measurements/Voltage Measurement  DialogController=POWERSYS.PowerSysDialog  SystemSampleTime=-1  PhasorSimulation=off  OutputType=Complex  PSBequivalent=0
  f-estimator : Subsystem  mask{dt=0.010}
      mask prompts: dt "sample time"
  load shedding logic : M-S-Function  FunctionName=load_shedding_logic3
  A : PMIOPort  Port=1  Side=Left
  B : PMIOPort  Port=2  Side=Left
  C : PMIOPort  Port=3  Side=Left
  w : Outport  OutDataType=fixdt(1, 16)  OutScaling=2^0
  state : Outport  Port=2  OutDataType=fixdt(1, 16)  OutScaling=2^0
  PQ : Outport  Port=3  OutDataType=fixdt(1, 16)  OutScaling=2^0
  V : Outport  Port=4  OutDataType=fixdt(1, 16)  OutScaling=2^0
  I : Outport  Port=5  OutDataType=fixdt(1, 16)  OutScaling=2^0
  RMS : Outport  Port=6  OutDataType=fixdt(1, 16)  OutScaling=2^0
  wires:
  reset/1 -> load shedding logic/1
  Current Measurement/1 -> RMS 1/1
  Voltage  Measurement/1 -> "RMS "/1, f-estimator/1(v)
  f-estimator/1(w) -> load shedding logic/2, w/1
  "RMS "/1 -> load shedding logic/3
  RMS 1/1 -> load shedding logic/4
  load shedding logic/1 -> Three-Phase Breaker2/1, state/1
  priority/1 -> load shedding logic/5
  Three-Phase V-I Measurement1/1 -> 3-phase  Instantaneous  Active & Reactive Power/1, RMS block1/1, V/1
  Three-Phase V-I Measurement1/2 -> 3-phase  Instantaneous  Active & Reactive Power/2, RMS block/1, I/1
  3-phase  Instantaneous  Active & Reactive Power/1 -> PQ/1
  RMS block1/1 -> Mux1/1
  RMS block/1 -> Mux1/2
  Mux1/1 -> RMS/1
  shed_load/1 -> load shedding logic/6
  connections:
  Voltage  Measurement/LConn1 -- Current Measurement/LConn1 -- Three-Phase V-I Measurement1/RConn1
  Voltage  Measurement/LConn2 -- Ground/LConn1
  Current Measurement/RConn1 -- Three-Phase Breaker2/LConn1
  L1/LConn1 -- Three-Phase Breaker2/RConn1
  L1/LConn2 -- Three-Phase Breaker2/RConn2
  L1/LConn3 -- Three-Phase Breaker2/RConn3
  Three-Phase V-I Measurement1/LConn1 -- A/RConn1
  Three-Phase V-I Measurement1/LConn2 -- B/RConn1
  Three-Phase V-I Measurement1/LConn3 -- C/RConn1
  Three-Phase V-I Measurement1/RConn2 -- Three-Phase Breaker2/LConn2
  Three-Phase V-I Measurement1/RConn3 -- Three-Phase Breaker2/LConn3

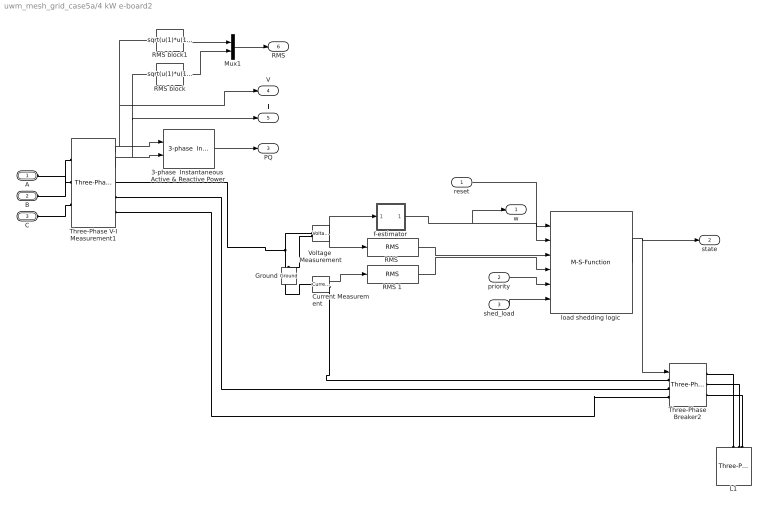
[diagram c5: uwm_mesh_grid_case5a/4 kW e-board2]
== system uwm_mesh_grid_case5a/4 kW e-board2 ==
  reset : Inport
  priority : Inport  Port=2
  shed_load : Inport  Port=3
  3-phase  Instantaneous  Active & Reactive Power : powerlib_extras/Measurements/3-phase  Instantaneous  Active & Reactive Power  DialogController=POWERSYS.PowerSysDialog  SystemSampleTime=-1
  Current Measurement : powerlib/Measurements/Current Measurement  DialogController=POWERSYS.PowerSysDialog  SystemSampleTime=-1  PhasorSimulation=off  OutputType=Complex  PSBequivalent=0
  Ground : powerlib/Elements/Ground  DialogController=POWERSYS.PowerSysDialog  PhysicalDomain=powersysdomain  SubClassName=unknown  LeftPortType=p1  RightPortType=p1  LConnTagsString=a
  L1 : powerlib/Elements/Three-Phase Series RLC Load  DialogController=POWERSYS.PowerSysDialog  PhysicalDomain=powersysdomain  SubClassName=unknown  LeftPortType=p1  RightPortType=p1  LConnTagsString=A|B|C  Configuration=Y (grounded)  NominalVoltage=208  NominalFrequency=60  ActivePower=4000  InductivePower=0  CapacitivePower=0  Measurements=None
  Mux1 : Mux  Inputs=2
  "RMS " : powerlib_extras/Measurements/RMS  DialogController=POWERSYS.PowerSysDialog  SystemSampleTime=-1  f1=60
  RMS 1 : powerlib_extras/Measurements/RMS  DialogController=POWERSYS.PowerSysDialog  SystemSampleTime=-1  f1=60
  RMS block : Fcn  Expr=sqrt(u(1)*u(1)+u(2)*u(2)+u(3)*u(3))/sqrt(3)
  RMS block1 : Fcn  Expr=sqrt(u(1)*u(1)+u(2)*u(2)+u(3)*u(3))/sqrt(3)
  Three-Phase V-I Measurement1 : powerlib/Measurements/Three-Phase V-I Measurement  DialogController=POWERSYS.PowerSysDialog  SystemSampleTime=-1  VoltageMeasurement=phase-to-ground  SetLabelV=off  LabelV=Vabc  Vpu=off  VpuLL=off  CurrentMeasurement=yes  SetLabelI=off  LabelI=Iabc  Ipu=off  Pbase=100e6  Vbase=500e3  OutputType=Complex  PhasorSimulation=off  PSBequivalent=0
  Three-Phase Breaker2 : powerlib/Elements/Three-Phase Breaker  DialogController=POWERSYS.PowerSysDialog  SystemSampleTime=-1  InitialState=closed  SwitchA=on  SwitchB=on  SwitchC=on  SwitchTimes=[50]  External=on  BreakerResistance=0.001  SnubberResistance=1e6  SnubberCapacitance=inf  Measurements=None
  Voltage  Measurement : powerlib/Measurements/Voltage Measurement  DialogController=POWERSYS.PowerSysDialog  SystemSampleTime=-1  PhasorSimulation=off  OutputType=Complex  PSBequivalent=0
  f-estimator : Subsystem  mask{dt=0.010}
      mask prompts: dt "sample time"
  load shedding logic : M-S-Function  FunctionName=load_shedding_logic3
  A : PMIOPort  Port=1  Side=Left
  B : PMIOPort  Port=2  Side=Left
  C : PMIOPort  Port=3  Side=Left
  w : Outport  OutDataType=fixdt(1, 16)  OutScaling=2^0
  state : Outport  Port=2  OutDataType=fixdt(1, 16)  OutScaling=2^0
  PQ : Outport  Port=3  OutDataType=fixdt(1, 16)  OutScaling=2^0
  V : Outport  Port=4  OutDataType=fixdt(1, 16)  OutScaling=2^0
  I : Outport  Port=5  OutDataType=fixdt(1, 16)  OutScaling=2^0
  RMS : Outport  Port=6  OutDataType=fixdt(1, 16)  OutScaling=2^0
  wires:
  reset/1 -> load shedding logic/1
  Current Measurement/1 -> RMS 1/1
  Voltage  Measurement/1 -> "RMS "/1, f-estimator/1(v)
  f-estimator/1(w) -> load shedding logic/2, w/1
  "RMS "/1 -> load shedding logic/3
  RMS 1/1 -> load shedding logic/4
  load shedding logic/1 -> Three-Phase Breaker2/1, state/1
  priority/1 -> load shedding logic/5
  Three-Phase V-I Measurement1/1 -> 3-phase  Instantaneous  Active & Reactive Power/1, RMS block1/1, V/1
  Three-Phase V-I Measurement1/2 -> 3-phase  Instantaneous  Active & Reactive Power/2, RMS block/1, I/1
  3-phase  Instantaneous  Active & Reactive Power/1 -> PQ/1
  RMS block1/1 -> Mux1/1
  RMS block/1 -> Mux1/2
  Mux1/1 -> RMS/1
  shed_load/1 -> load shedding logic/6
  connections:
  Voltage  Measurement/LConn1 -- Current Measurement/LConn1 -- Three-Phase V-I Measurement1/RConn1
  Voltage  Measurement/LConn2 -- Ground/LConn1
  Current Measurement/RConn1 -- Three-Phase Breaker2/LConn1
  L1/LConn1 -- Three-Phase Breaker2/RConn1
  L1/LConn2 -- Three-Phase Breaker2/RConn2
  L1/LConn3 -- Three-Phase Breaker2/RConn3
  Three-Phase V-I Measurement1/LConn1 -- A/RConn1
  Three-Phase V-I Measurement1/LConn2 -- B/RConn1
  Three-Phase V-I Measurement1/LConn3 -- C/RConn1
  Three-Phase V-I Measurement1/RConn2 -- Three-Phase Breaker2/LConn2
  Three-Phase V-I Measurement1/RConn3 -- Three-Phase Breaker2/LConn3
